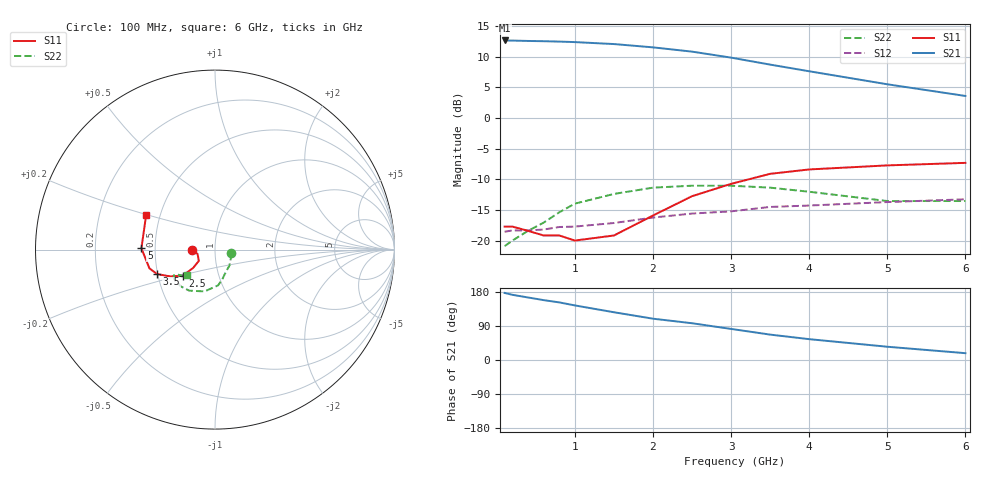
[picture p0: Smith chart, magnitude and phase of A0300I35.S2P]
!  MSA-0300 S AND NOISE PARAMETERS
!  Id=35mA  LAST UPDATED 07-22-92
# ghz s ma r 50
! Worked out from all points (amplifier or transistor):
!   14 points, 100 MHz to 6 GHz, reference 50 ohm
!   highest |S21| = 12.6 dB at 100 MHz (marker M1)
!   |S21| within 3 dB of that: start of sweep to 3.087 GHz
!   unconditionally stable (mu >= 1): start of sweep to 2.423 GHz; 3.853 GHz to end of sweep
!   at 400 MHz: K = 1.19, MAG = 12.8 dB, |S12| = -18.3 dB
!   at 2 GHz: K = 1.03, MAG = 12.8 dB, |S12| = -16.2 dB
!   at 6 GHz: K = 1.27, MAG = 5.3 dB, |S12| = -13.3 dB
!   lowest NFmin = 5.50 dB at 100 MHz
!   S11 on the Smith chart (normalised r, x): 100 MHz: 0.77, -0.00; 2.5 GHz: 0.67, -0.21; 3.5 GHz: 0.50, -0.15; 5 GHz: 0.42, +0.01; 6 GHz: 0.42, +0.20
0.1  0.13 -179.0  4.28 177.0  0.118 2.0  0.09 -13.0
0.2  0.13 -179.0  4.27 172.0  0.121 3.0  0.1 -27.0
0.4  0.12 -179.0  4.24 165.0  0.121 5.0  0.12 -48.0
0.6  0.11 -177.0  4.22 158.0  0.123 8.0  0.14 -65.0
0.8  0.11 -172.0  4.19 152.0  0.129 11.0  0.17 -76.0
1  0.1 -166.0  4.15 144.0  0.13 12.0  0.2 -85.0
1.5  0.11 -145.0  4 126.0  0.139 17.0  0.24 -104.0
2  0.16 -140.0  3.76 109.0  0.154 20.0  0.27 -122.0
2.5  0.23 -141.0  3.47 97.0  0.166 25.0  0.28 -133.0
3  0.29 -149.0  3.1 82.0  0.173 24.0  0.28 -145.0
3.5  0.35 -157.0  2.72 67.0  0.188 22.0  0.27 -148.0
4  0.38 -164.0  2.4 55.0  0.193 21.0  0.25 -146.0
5  0.41 179.0  1.88 35.0  0.206 17.0  0.21 -134.0
6  0.43 153.0  1.51 18.0  0.217 14.0  0.21 -137.0
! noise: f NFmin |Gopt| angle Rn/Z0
0.1  5.5  0.04  1  0.82
0.5  5.8  0.04  12  0.82
1  6  0.03  15  0.81
2  6.5  0.01  128  0.79
